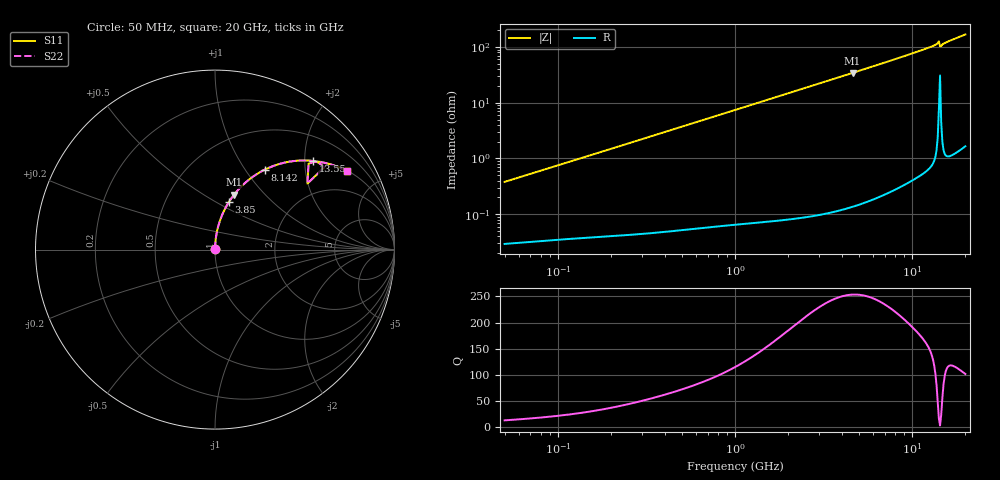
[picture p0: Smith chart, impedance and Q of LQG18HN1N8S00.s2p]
!Murata Part Number: LQG18HN1N8S00
!These Parameters are Measured in Series Mode Connection
!  o--[Z]--o
!Port1  Port2
!  o-------o
!Freq. Start=50[MHz] Stop=20[GHz], 401[Steps]
# Hz S RI R 50
!Freq.(Hz) S11(Real) S11(Imag) S21(Real) S21(Imag) S12(Real) S12(Imag) S22(Real) S22(Imag)
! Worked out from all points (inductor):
!   401 points, 50 MHz to 20 GHz, reference 50 ohm
!   read as one part in series: L = 1.2 nH near 51.52 MHz
!   highest Q = 253 at 4.608 GHz (marker M1), where L = 1.19 nH
!   S11 on the Smith chart (normalised r, x): 50 MHz: 1.00, +0.01; 3.85 GHz: 1.00, +0.57; 8.142 GHz: 1.01, +1.23; 13.55 GHz: 1.02, +2.20; 20 GHz: 1.03, +3.37
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5e7  0.000307 0.00379  0.9997 -0.00379  0.9997 -0.00379  0.000307 0.00379
1.364002e8  0.000477 0.0102  0.9995 -0.0102  0.9995 -0.0102  0.000477 0.0102
3.721004e8  0.00124 0.0277  0.9988 -0.0277  0.9988 -0.0277  0.00124 0.0277
6.380365e8  0.0028 0.0472  0.9972 -0.0472  0.9972 -0.0472  0.0028 0.0472
1e9  0.00611 0.0737  0.9939 -0.0737  0.9939 -0.0737  0.00611 0.0737
1.689197e9  0.0162 0.1231  0.9838 -0.1231  0.9838 -0.1231  0.0162 0.1231
2.728004e9  0.0402 0.1941  0.9598 -0.1941  0.9598 -0.1941  0.0402 0.1941
3.850025e9  0.0767 0.2641  0.9233 -0.2641  0.9233 -0.2641  0.0767 0.2641
4.608136e9  0.1065 0.3065  0.8935 -0.3065  0.8935 -0.3065  0.1065 0.3065
5.856089e9  0.1623 0.3667  0.8377 -0.3667  0.8377 -0.3667  0.1623 0.3667
7.442007e9  0.2406 0.4253  0.7594 -0.4253  0.7594 -0.4253  0.2406 0.4253
8.141811e9  0.2764 0.4449  0.7236 -0.4449  0.7236 -0.4449  0.2764 0.4449
1.082228e10  0.412 0.4894  0.588 -0.4894  0.588 -0.4894  0.412 0.4894
1.257102e10  0.4962 0.4966  0.5038 -0.4966  0.5038 -0.4966  0.4962 0.4966
1.354865e10  0.5465 0.4929  0.4535 -0.4929  0.4535 -0.4929  0.5465 0.4929
1.375312e10  0.56 0.4901  0.44 -0.4901  0.44 -0.4901  0.56 0.4901
1.396067e10  0.5781 0.4837  0.4219 -0.4837  0.4219 -0.4837  0.5781 0.4837
1.482269e10  0.5514 0.4884  0.4486 -0.4884  0.4486 -0.4884  0.5514 0.4884
1.504638e10  0.5689 0.4891  0.4311 -0.4891  0.4311 -0.4891  0.5689 0.4891
1.550395e10  0.5934 0.4866  0.4066 -0.4866  0.4066 -0.4866  0.5934 0.4866
1.774144e10  0.6745 0.4642  0.3255 -0.4642  0.3255 -0.4642  0.6745 0.4642
2e10  0.7374 0.4352  0.2626 -0.4352  0.2626 -0.4352  0.7374 0.4352
